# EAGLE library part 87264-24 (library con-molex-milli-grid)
RECEPTACAL
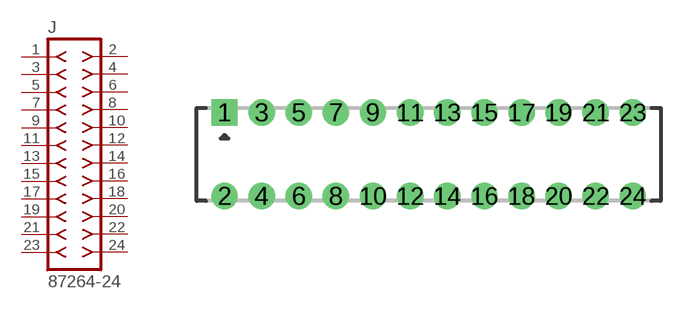
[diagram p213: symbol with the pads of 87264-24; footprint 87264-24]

Designator prefix J

## 87264-24  [87264-24]
1  1  pas
2  2  pas
3  3  pas
4  4  pas
5  5  pas
6  6  pas
7  7  pas
8  8  pas
9  9  pas
10  10  pas
11  11  pas
12  12  pas
13  13  pas
14  14  pas
15  15  pas
16  16  pas
17  17  pas
18  18  pas
19  19  pas
20  20  pas
21  21  pas
22  22  pas
23  23  pas
24  24  pas

## Footprint 87264-24 (pad centres in mm)
RECEPTACAL Dual Row, Side Entry
drill 0.914 square: 1 -11,2.25
drill 0.914: 2 -11,-2.25; 3 -9,2.25; 4 -9,-2.25; 5 -7,2.25; 6 -7,-2.25; 7 -5,2.25; 8 -5,-2.25; 9 -3,2.25; 10 -3,-2.25; 11 -1,2.25; 12 -1,-2.25; 13 1,2.25; 14 1,-2.25; 15 3,2.25; 16 3,-2.25; 17 5,2.25; 18 5,-2.25; 19 7,2.25; 20 7,-2.25; 21 9,2.25; 22 9,-2.25; 23 11,2.25; 24 11,-2.25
